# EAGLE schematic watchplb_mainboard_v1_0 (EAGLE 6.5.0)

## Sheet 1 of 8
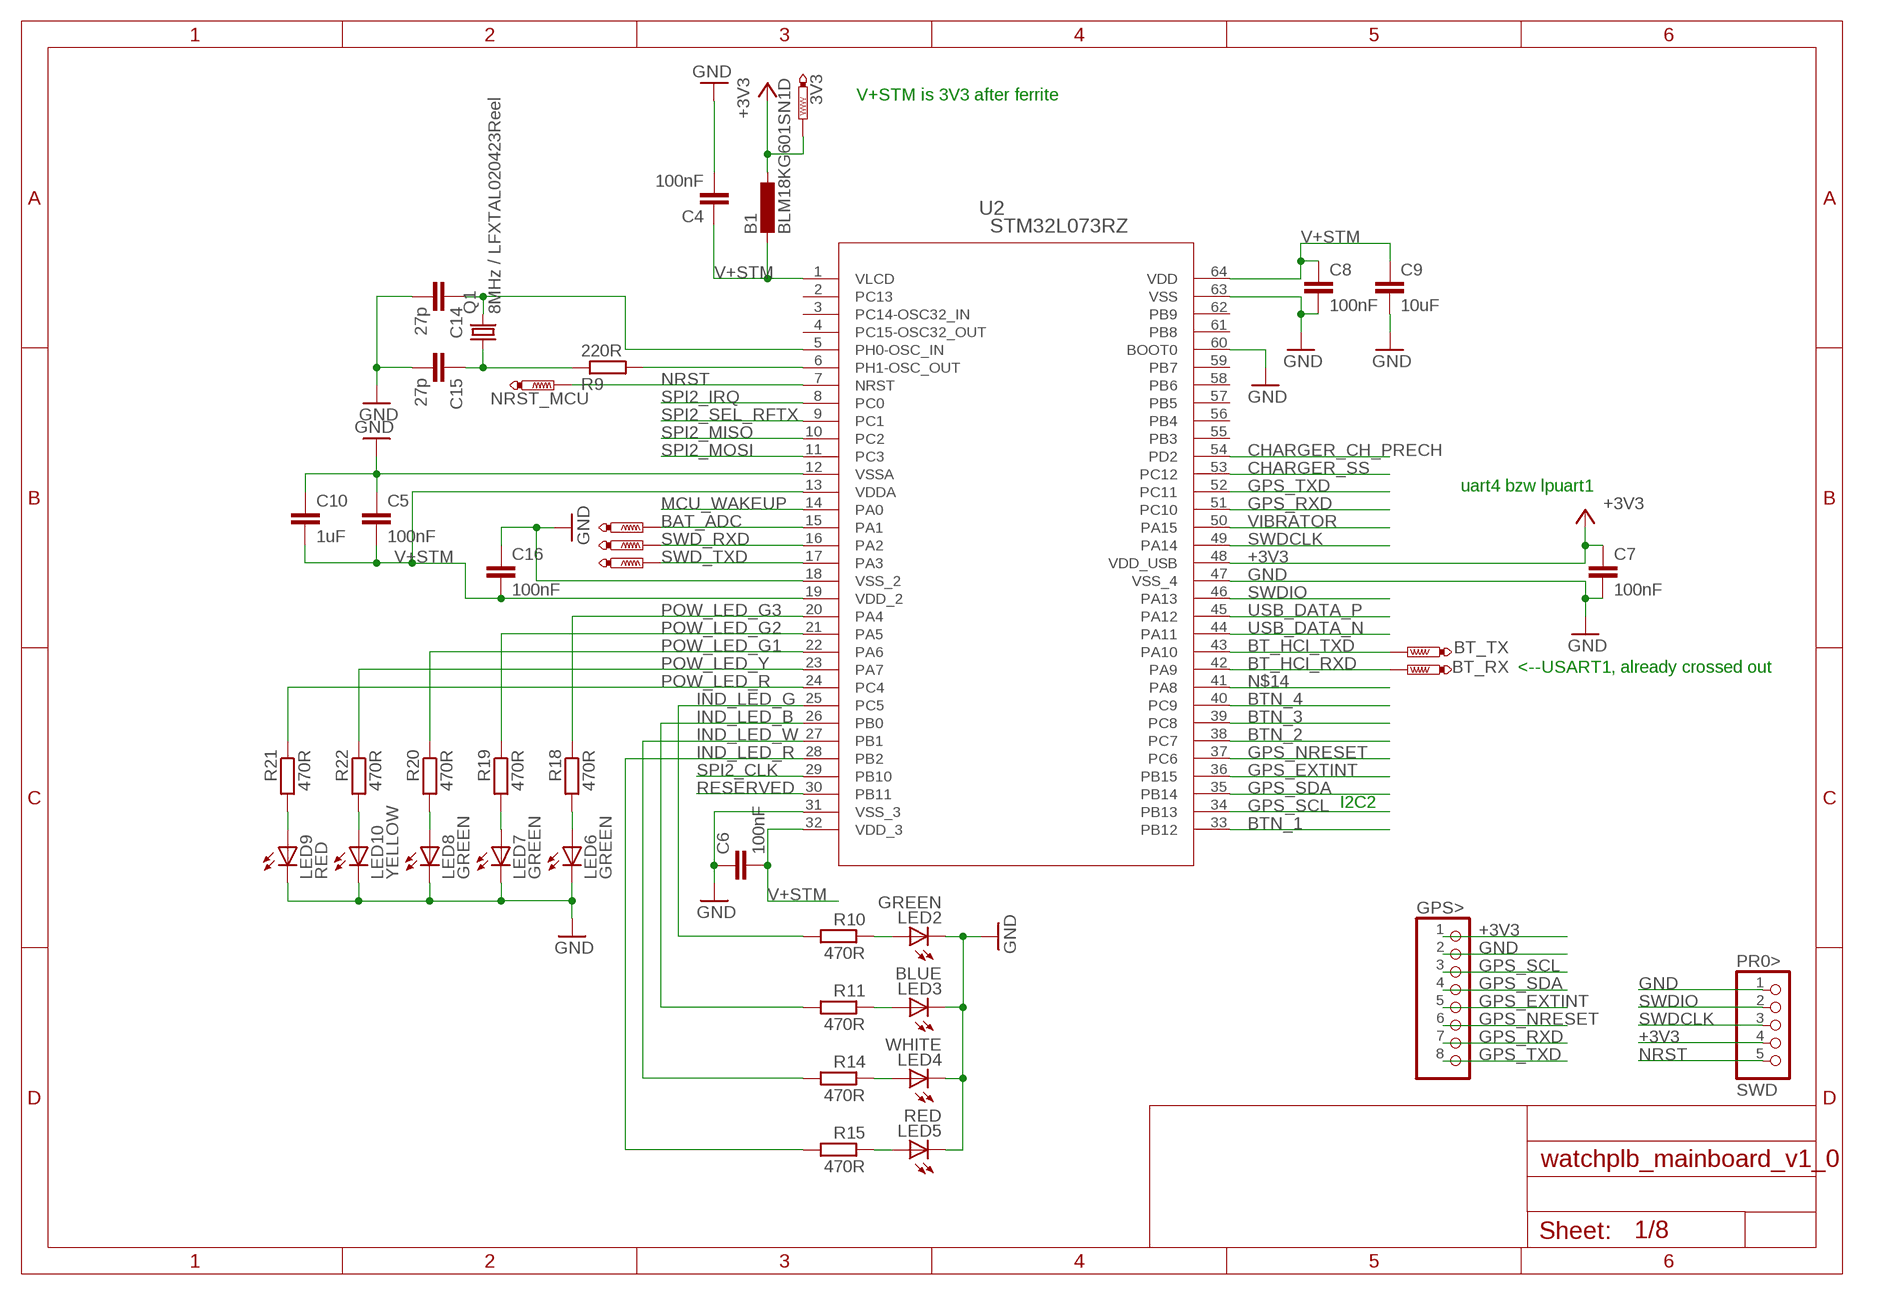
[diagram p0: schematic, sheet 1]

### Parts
3V3  PTR1B1,27  [B1,27]
B1  BLM18KG601SN1D  B-EU_B0603  [L0603]
BAT_ADC  PTR1B1,27  [B1,27]
BT_RX  PTR1B1,27  [B1,27]
BT_TX  PTR1B1,27  [B1,27]
C4  100nF  C-EUC0805  [C0805]
C5  100nF  C-EUC0805  [C0805]
C6  100nF  C-EUC0805  [C0805]
C7  100nF  C-EUC0805  [C0805]
C8  100nF  C-EUC0805  [C0805]
C9  10uF  C-EUC1206  [C1206]
C10  1uF  C-EUC0805  [C0805]
C14  27p  C-EUC0805  [C0805]
C15  27p  C-EUC0805  [C0805]
C16  100nF  C-EUC0805  [C0805]
GPS>  PINHD-1X8  [1X08]
LED2  GREEN  LEDCHIP-LED0805  [CHIP-LED0805]
LED3  BLUE  LEDCHIP-LED0805  [CHIP-LED0805]
LED4  WHITE  LEDCHIP-LED0805  [CHIP-LED0805]
LED5  RED  LEDCHIP-LED0805  [CHIP-LED0805]
LED6  GREEN  LEDCHIP-LED0805  [CHIP-LED0805]
LED7  GREEN  LEDCHIP-LED0805  [CHIP-LED0805]
LED8  GREEN  LEDCHIP-LED0805  [CHIP-LED0805]
LED9  RED  LEDCHIP-LED0805  [CHIP-LED0805]
LED10  YELLOW  LEDCHIP-LED0805  [CHIP-LED0805]
NRST_MCU  PTR1B1,27  [B1,27]
PR0>  SWD  PINHD-1X5  [1X05]
Q1  8MHz / LFXTAL020423Reel  CRYSTALHC49UP  [HC49UP]
R9  220R  R-EU_M0805  [M0805]
R10  470R  R-EU_M0805  [M0805]
R11  470R  R-EU_M0805  [M0805]
R14  470R  R-EU_M0805  [M0805]
R15  470R  R-EU_M0805  [M0805]
R18  470R  R-EU_M0805  [M0805]
R19  470R  R-EU_M0805  [M0805]
R20  470R  R-EU_M0805  [M0805]
R21  470R  R-EU_M0805  [M0805]
R22  470R  R-EU_M0805  [M0805]
SWD_RXD  PTR1B1,27  [B1,27]
SWD_TXD  PTR1B1,27  [B1,27]
U2  STM32L073RZ  STM32L0X3RL  [LQFP64-10X10MM]

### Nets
+3V3: 3V3.TP B1.1 C7.1 GPS>.1 PR0>.4 U2.48(VDD_USB) ; also sheet 2,3,4,5,6,8
BAT_ADC: BAT_ADC.TP U2.15(PA1) ; also sheet 8
BT_HCI_RXD: BT_RX.TP U2.42(PA9) ; also sheet 4
BT_HCI_TXD: BT_TX.TP U2.43(PA10) ; also sheet 4
BTN_1: U2.33(PB12) ; also sheet 3
BTN_2: U2.38(PC7) ; also sheet 3
BTN_3: U2.39(PC8) ; also sheet 3
BTN_4: U2.40(PC9) ; also sheet 3
CHARGER_CH_PRECH: U2.54(PD2) ; also sheet 5
CHARGER_SS: U2.53(PC12) ; also sheet 5
GND: C4.2 C5.1 C6.1 C7.2 C8.2 C9.2 C10.1 C14.2 C15.2 C16.1 GPS>.2 LED2.C LED3.C LED4.C LED5.C LED6.C LED7.C LED8.C LED9.C LED10.C PR0>.1 U2.12(VSSA) U2.18(VSS_2) U2.31(VSS_3) U2.47(VSS_4) U2.60(BOOT0) U2.63(VSS) ; also sheet 2,3,4,5,6,7,8
GPS_EXTINT: GPS>.5 U2.36(PB15)
GPS_NRESET: GPS>.6 U2.37(PC6)
GPS_RXD: GPS>.7 U2.51(PC10)
GPS_SCL: GPS>.3 U2.34(PB13)
GPS_SDA: GPS>.4 U2.35(PB14)
GPS_TXD: GPS>.8 U2.52(PC11)
IND_LED_B: R11.2 U2.26(PB0)
IND_LED_G: R10.2 U2.25(PC5)
IND_LED_R: R15.2 U2.28(PB2)
IND_LED_W: R14.2 U2.27(PB1)
MCU_WAKEUP: U2.14(PA0) ; also sheet 3
N$1: LED2.A R10.1
N$4: LED3.A R11.1
N$5: C15.1 Q1.1 R9.1
N$6: C14.1 Q1.2 U2.5(PH0-OSC_IN)
N$9: R9.2 U2.6(PH1-OSC_OUT)
N$12: LED4.A R14.1
N$13: LED9.A R21.2
N$14: U2.41(PA8)
N$16: LED5.A R15.1
N$19: LED6.A R18.2
N$22: LED7.A R19.2
N$24: LED10.A R22.2
N$25: LED8.A R20.2
NRST: NRST_MCU.TP PR0>.5 U2.7(NRST) ; also sheet 3
POW_LED_G1: R20.1 U2.22(PA6)
POW_LED_G2: R19.1 U2.21(PA5)
POW_LED_G3: R18.1 U2.20(PA4)
POW_LED_R: R21.1 U2.24(PC4)
POW_LED_Y: R22.1 U2.23(PA7)
RESERVED: U2.30(PB11)
SPI2_CLK: U2.29(PB10) ; also sheet 2
SPI2_IRQ: U2.8(PC0) ; also sheet 2
SPI2_MISO: U2.10(PC2) ; also sheet 2
SPI2_MOSI: U2.11(PC3) ; also sheet 2
SPI2_SEL_RFTX: U2.9(PC1) ; also sheet 2
SWD_RXD: SWD_RXD.TP U2.16(PA2)
SWD_TXD: SWD_TXD.TP U2.17(PA3)
SWDCLK: PR0>.3 U2.49(PA14)
SWDIO: PR0>.2 U2.46(PA13)
USB_DATA_N: U2.44(PA11) ; also sheet 6
USB_DATA_P: U2.45(PA12) ; also sheet 6
V+STM: B1.2 C4.1 C5.2 C6.2 C8.1 C9.1 C10.2 C16.2 U2.1(VLCD) U2.13(VDDA) U2.19(VDD_2) U2.32(VDD_3) U2.64(VDD)
VIBRATOR: U2.50(PA15) ; also sheet 3
Unconnected: U2.2(PC13) U2.3(PC14-OSC32_IN) U2.4(PC15-OSC32_OUT) U2.55(PB3) U2.56(PB4) U2.57(PB5) U2.58(PB6) U2.59(PB7) U2.61(PB8) U2.62(PB9)

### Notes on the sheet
- V+STM is 3V3 after ferrite
- uart4 bzw lpuart1
- <--USART1, already crossed out
- I2C2

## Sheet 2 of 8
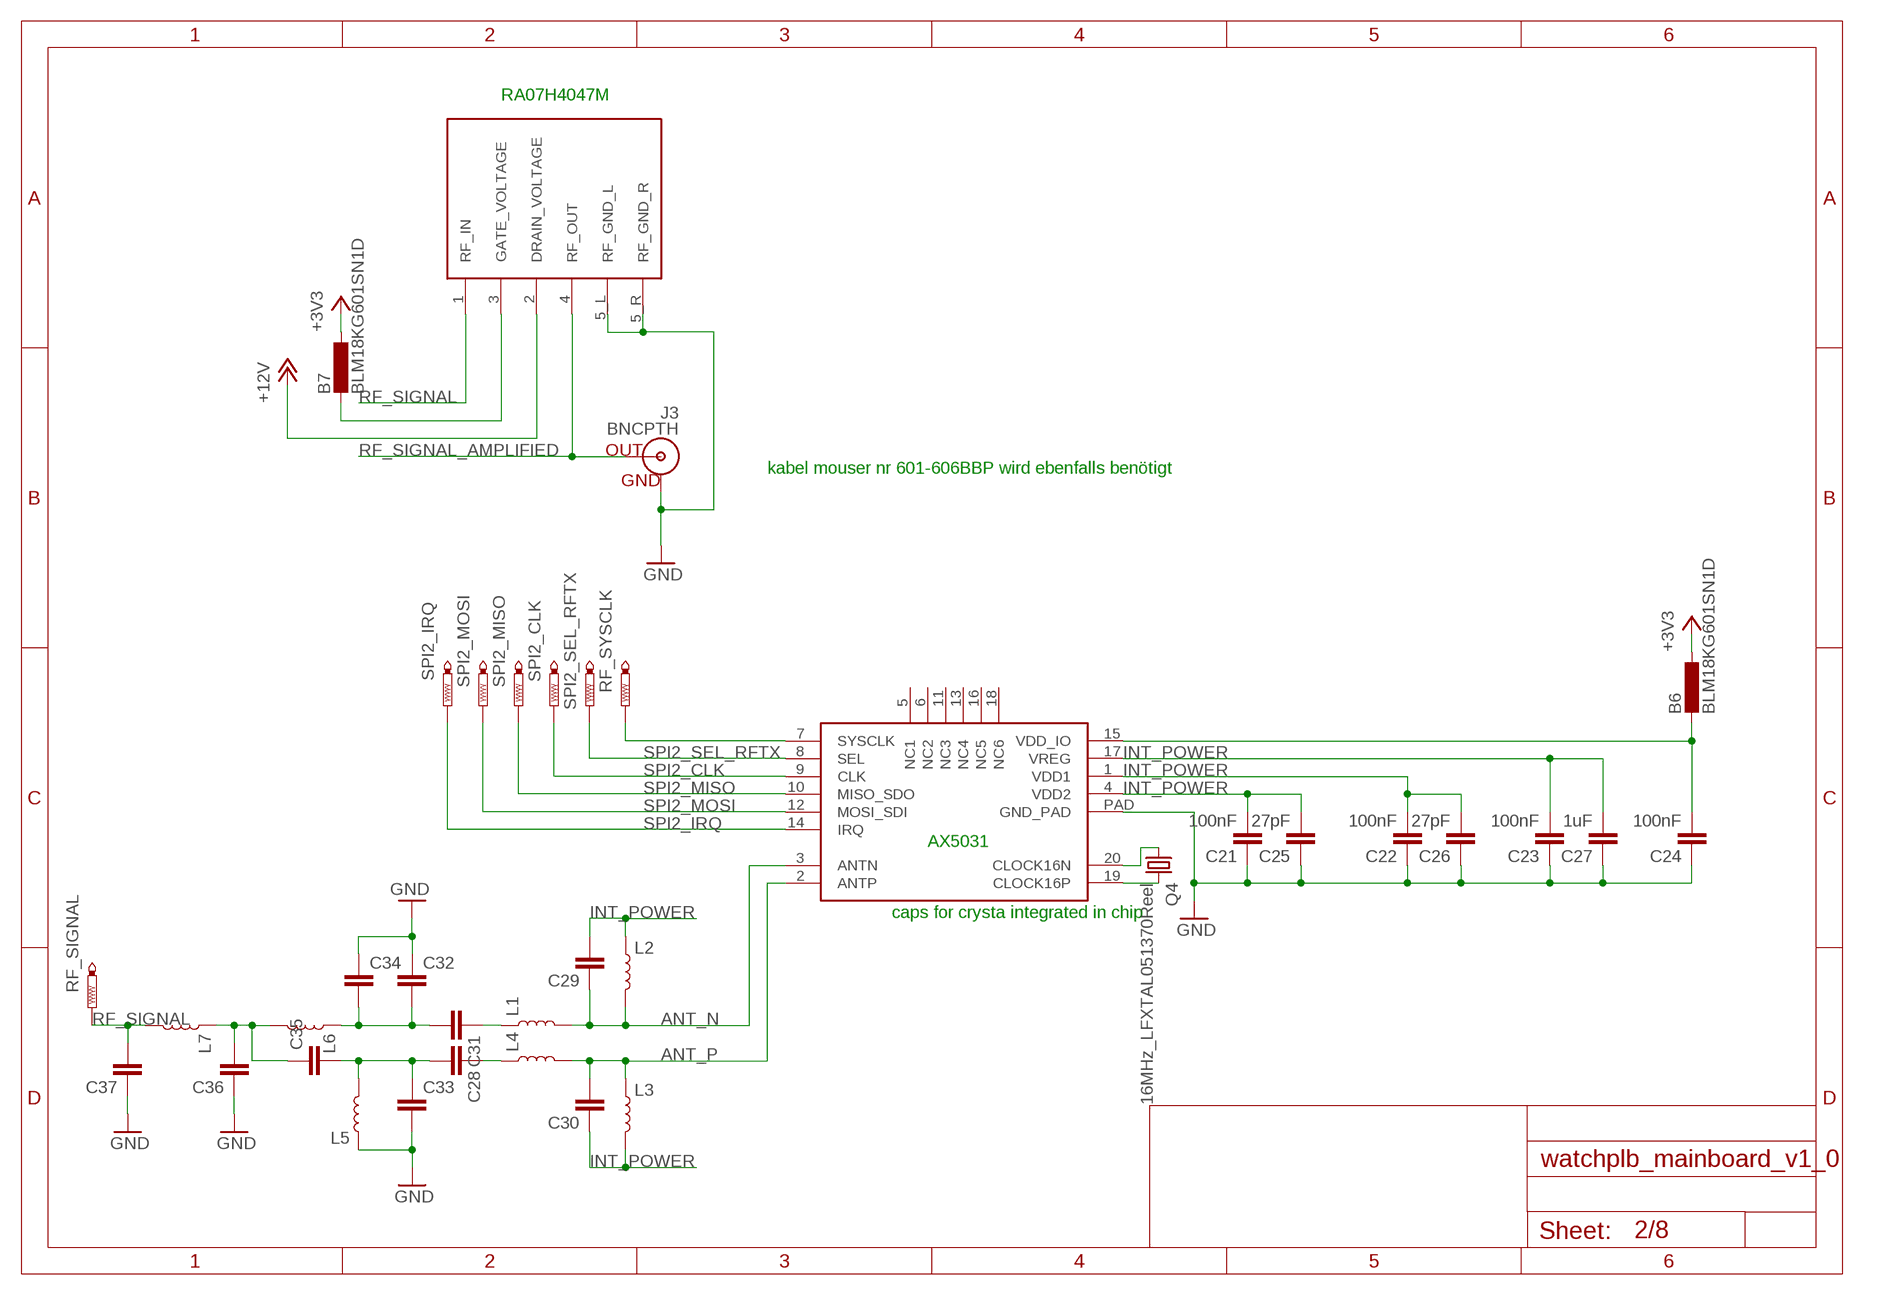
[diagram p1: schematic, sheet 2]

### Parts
B6  BLM18KG601SN1D  B-EU_B0603  [L0603]
B7  BLM18KG601SN1D  B-EU_B0603  [L0603]
C21  100nF  C-EUC0805  [C0805]
C22  100nF  C-EUC0805  [C0805]
C23  100nF  C-EUC0805  [C0805]
C24  100nF  C-EUC0805  [C0805]
C25  27pF  C-EUC0805  [C0805]
C26  27pF  C-EUC0805  [C0805]
C27  1uF  C-EUC0805  [C0805]
C28  C-EUC0805  [C0805]
C29  C-EUC0805  [C0805]
C30  C-EUC0805  [C0805]
C31  C-EUC0805  [C0805]
C32  C-EUC0805  [C0805]
C33  C-EUC0805  [C0805]
C34  C-EUC0805  [C0805]
C35  C-EUC0805  [C0805]
C36  C-EUC0805  [C0805]
C37  C-EUC0805  [C0805]
IC4  AX5031  [QFN20]
J3  BNCPTH  [BNC]
L1  INDUCTOR-0805-3.3UH  [0805]
L2  INDUCTOR-0805-3.3UH  [0805]
L3  INDUCTOR-0805-3.3UH  [0805]
L4  INDUCTOR-0805-3.3UH  [0805]
L5  INDUCTOR-0805-3.3UH  [0805]
L6  INDUCTOR-0805-3.3UH  [0805]
L7  INDUCTOR-0805-3.3UH  [0805]
Q4  16MHz_LFXTAL051370Reel  CRYSTALHC49UP  [HC49UP]
RF_SIGNAL  PTR1B2,54  [B2,54]
RF_SYSCLK  PTR1B1,27  [B1,27]
SPI2_CLK  PTR1B1,27  [B1,27]
SPI2_IRQ  PTR1B1,27  [B1,27]
SPI2_MISO  PTR1B1,27  [B1,27]
SPI2_MOSI  PTR1B1,27  [B1,27]
SPI2_SEL_RFTX  PTR1B1,27  [B1,27]
U$2  RA07H4047M  [RA07H4047M]

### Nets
+3V3: B6.1 B7.1 ; also sheet 1,3,4,5,6,8
+12V: U$2.2(DRAIN_VOLTAGE) ; also sheet 8
ANT_N: C29.1 IC4.3(ANTN) L1.2 L2.2
ANT_P: C30.2 IC4.2(ANTP) L3.1 L4.2
GND: C21.1 C22.1 C23.1 C24.1 C25.1 C26.1 C27.1 C32.1 C33.2 C34.1 C36.1 C37.1 IC4.PAD(GND_PAD) J3.GND L5.1 U$2.5_L(RF_GND_L) U$2.5_R(RF_GND_R) ; also sheet 1,3,4,5,6,7,8
INT_POWER: C21.2 C22.2 C23.2 C25.2 C26.2 C27.2 C29.2 C30.1 IC4.1(VDD1) IC4.4(VDD2) IC4.17(VREG) L2.1 L3.2
N$33: IC4.19(CLOCK16P) Q4.2
N$34: IC4.20(CLOCK16N) Q4.1
N$37: IC4.7(SYSCLK) RF_SYSCLK.TP
N$39: C28.1 L4.1
N$40: C31.1 L1.1
N$42: C31.2 C32.2 C34.2 L6.1
N$43: C28.2 C33.1 C35.2 L5.2
N$45: C35.1 C36.2 L6.2 L7.1
N$82: B6.2 C24.2 IC4.15(VDD_IO)
N$83: B7.2 U$2.3(GATE_VOLTAGE)
RF_SIGNAL: C37.2 L7.2 RF_SIGNAL.TP U$2.1(RF_IN)
RF_SIGNAL_AMPLIFIED: J3.S(OUT) U$2.4(RF_OUT)
SPI2_CLK: IC4.9(CLK) SPI2_CLK.TP ; also sheet 1
SPI2_IRQ: IC4.14(IRQ) SPI2_IRQ.TP ; also sheet 1
SPI2_MISO: IC4.10(MISO_SDO) SPI2_MISO.TP ; also sheet 1
SPI2_MOSI: IC4.12(MOSI_SDI) SPI2_MOSI.TP ; also sheet 1
SPI2_SEL_RFTX: IC4.8(SEL) SPI2_SEL_RFTX.TP ; also sheet 1
Unconnected: IC4.5(NC1) IC4.6(NC2) IC4.11(NC3) IC4.13(NC4) IC4.16(NC5) IC4.18(NC6)

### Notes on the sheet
- RA07H4047M
- kabel mouser nr 601-606BBP wird ebenfalls benötigt
- AX5031
- caps for crysta integrated in chip

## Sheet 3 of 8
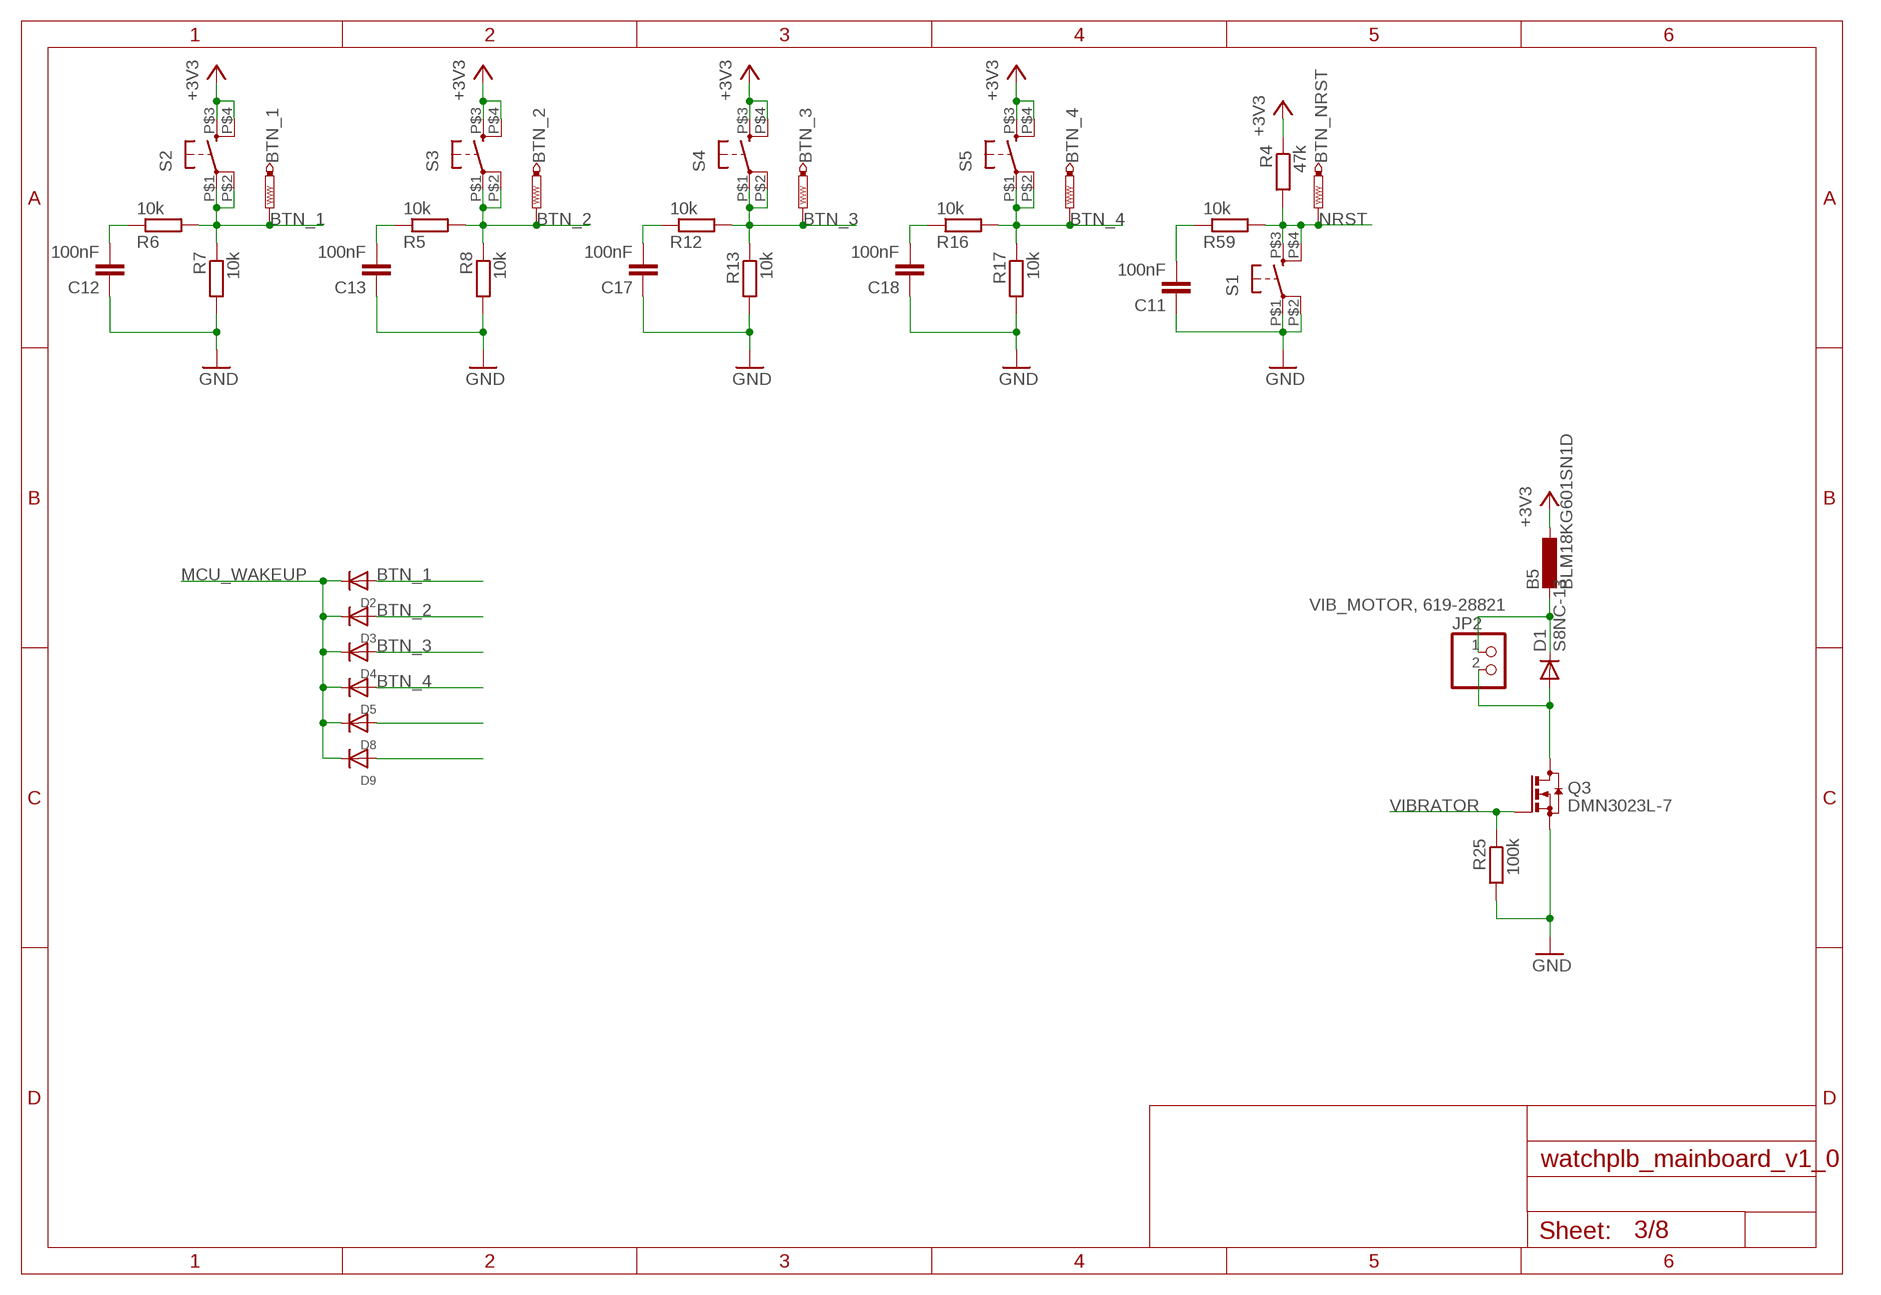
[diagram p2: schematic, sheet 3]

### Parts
B5  BLM18KG601SN1D  B-EU_B0603  [L0603]
BTN_1  PTR1B1,27  [B1,27]
BTN_2  PTR1B1,27  [B1,27]
BTN_3  PTR1B1,27  [B1,27]
BTN_4  PTR1B1,27  [B1,27]
BTN_NRST  PTR1B1,27  [B1,27]
C11  100nF  C-EUC0805  [C0805]
C12  100nF  C-EUC0805  [C0805]
C13  100nF  C-EUC0805  [C0805]
C17  100nF  C-EUC0805  [C0805]
C18  100nF  C-EUC0805  [C0805]
D1  S8NC-13  DIODE-SMC  [SMC]
D2  DIODESOD-123  [SOD-123]
D3  DIODESOD-123  [SOD-123]
D4  DIODESOD-123  [SOD-123]
D5  DIODESOD-123  [SOD-123]
D8  DIODESOD-123  [SOD-123]
D9  DIODESOD-123  [SOD-123]
JP2  VIB_MOTOR, 619-28821  PINHD-1X2  [1X02]
Q3  DMN3023L-7  BSS123  [SOT23]
R4  47k  R-EU_M0805  [M0805]
R5  10k  R-EU_M0805  [M0805]
R6  10k  R-EU_M0805  [M0805]
R7  10k  R-EU_M0805  [M0805]
R8  10k  R-EU_M0805  [M0805]
R12  10k  R-EU_M0805  [M0805]
R13  10k  R-EU_M0805  [M0805]
R16  10k  R-EU_M0805  [M0805]
R17  10k  R-EU_M0805  [M0805]
R25  100k  R-EU_M0805  [M0805]
R59  10k  R-EU_M0805  [M0805]
S1  TL3305  [SMD_SWITCH]
S2  TL3305  [SMD_SWITCH]
S3  TL3305  [SMD_SWITCH]
S4  TL3305  [SMD_SWITCH]
S5  TL3305  [SMD_SWITCH]

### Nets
+3V3: B5.1 R4.1 S2.P$3(S) S2.P$4(S1) S3.P$3(S) S3.P$4(S1) S4.P$3(S) S4.P$4(S1) S5.P$3(S) S5.P$4(S1) ; also sheet 1,2,4,5,6,8
BTN_1: BTN_1.TP D2.A R6.2 R7.1 S2.P$1(P) S2.P$2(P1) ; also sheet 1
BTN_2: BTN_2.TP D3.A R5.2 R8.1 S3.P$1(P) S3.P$2(P1) ; also sheet 1
BTN_3: BTN_3.TP D4.A R12.2 R13.1 S4.P$1(P) S4.P$2(P1) ; also sheet 1
BTN_4: BTN_4.TP D5.A R16.2 R17.1 S5.P$1(P) S5.P$2(P1) ; also sheet 1
GND: C11.1 C12.1 C13.1 C17.1 C18.1 Q3.2(S) R7.2 R8.2 R13.2 R17.2 R25.2 S1.P$1(P) S1.P$2(P1) ; also sheet 1,2,4,5,6,7,8
MCU_WAKEUP: D2.C D3.C D4.C D5.C D8.C D9.C ; also sheet 1
N$2: C12.2 R6.1
N$7: C13.2 R5.1
N$11: C17.2 R12.1
N$18: C18.2 R16.1
N$28: D1.A JP2.2 Q3.3(D)
N$67: D8.A
N$68: D9.A
N$81: B5.2 D1.C JP2.1
N$86: C11.2 R59.1
NRST: BTN_NRST.TP R4.2 R59.2 S1.P$3(S) S1.P$4(S1) ; also sheet 1
VIBRATOR: Q3.1(G) R25.1 ; also sheet 1

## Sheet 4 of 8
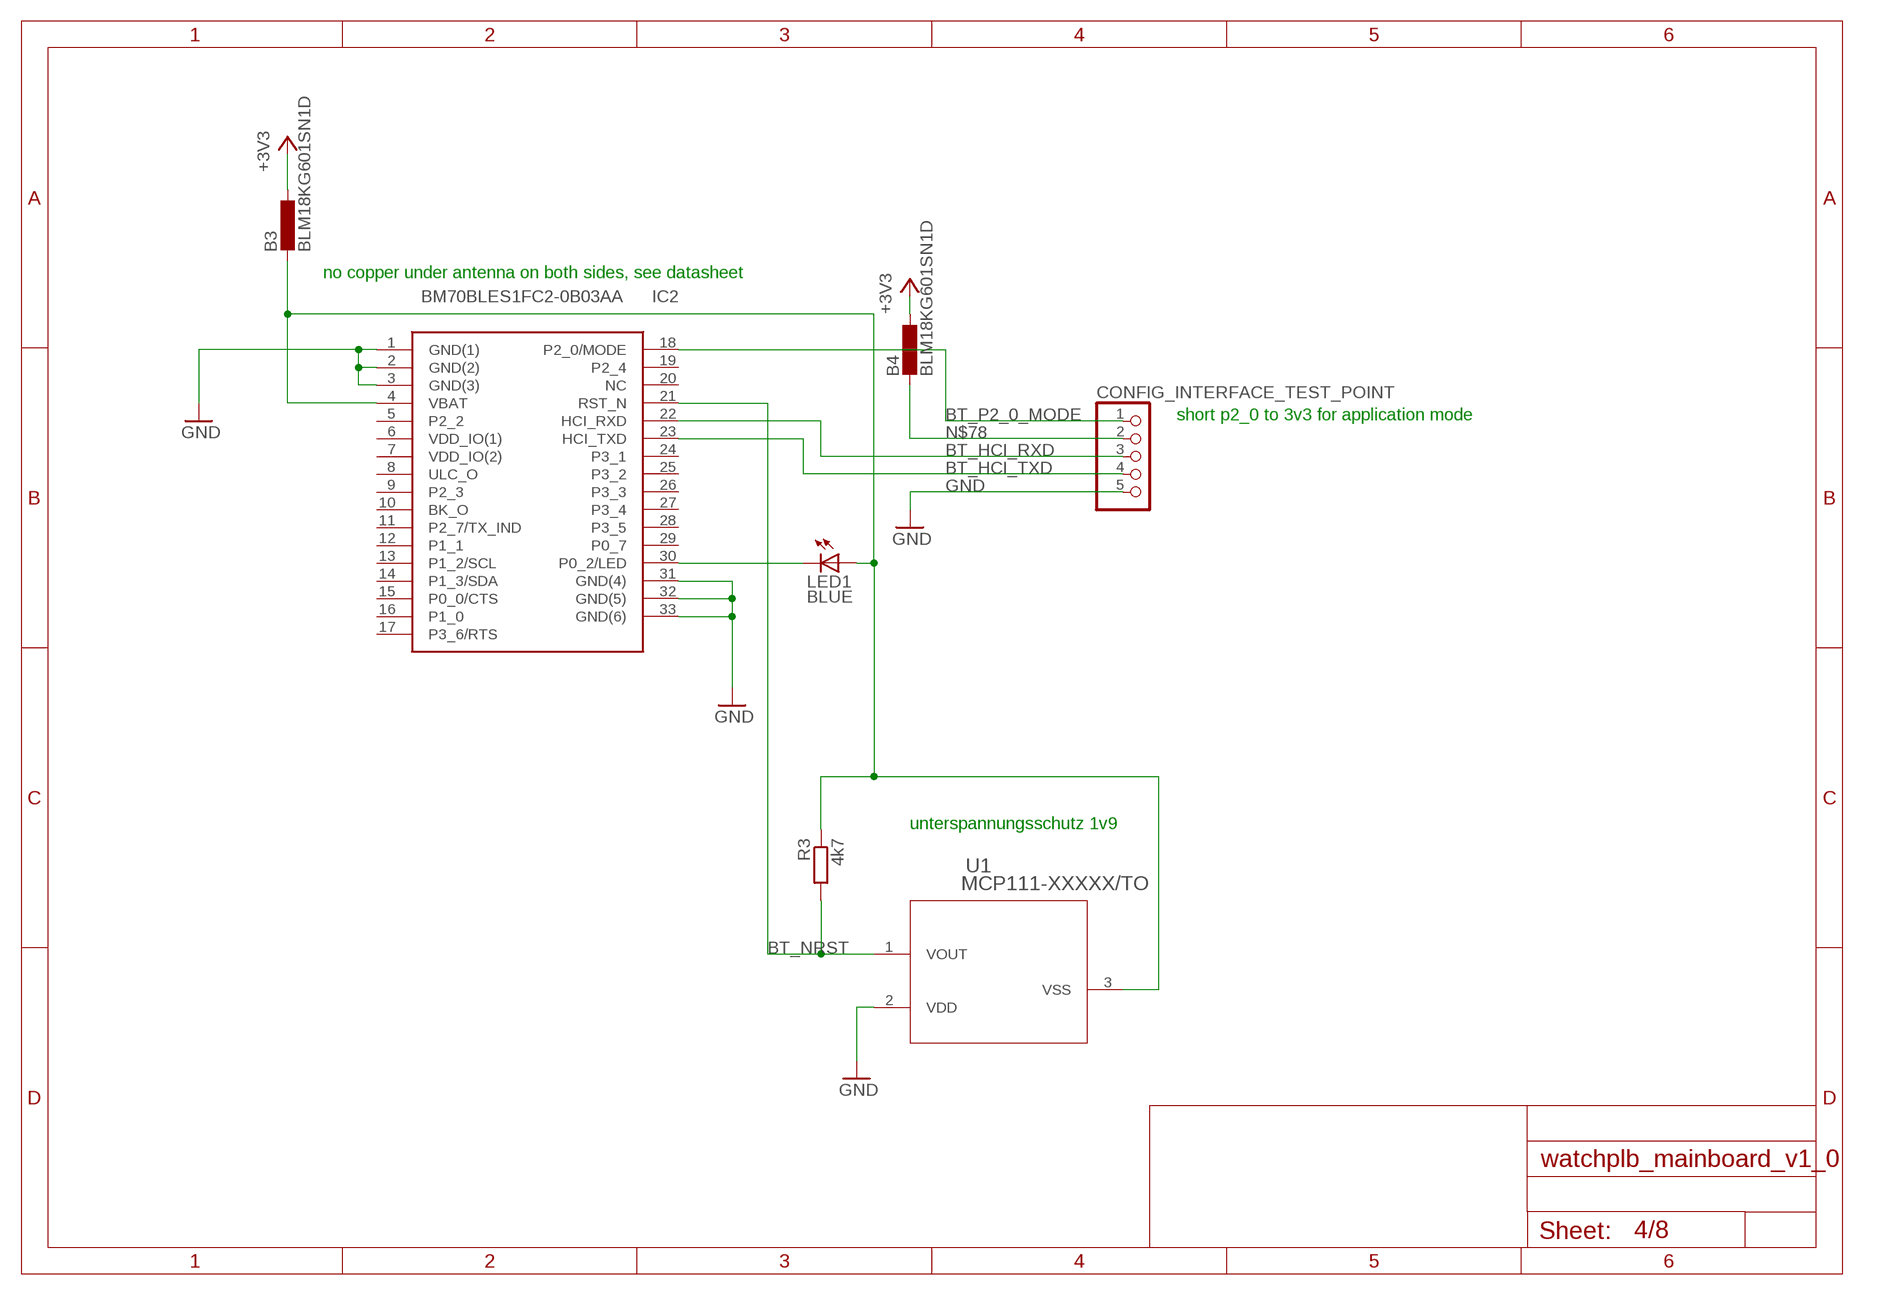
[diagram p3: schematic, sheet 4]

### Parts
B3  BLM18KG601SN1D  B-EU_B0603  [L0603]
B4  BLM18KG601SN1D  B-EU_B0603  [L0603]
CONFIG_INTERFACE_TEST_POINT  PINHD-1X5  [1X05]
IC2  BM70BLES1FC2-0B03AA  [BM78SPPS5NC2_1]
LED1  BLUE  LEDCHIP-LED0805  [CHIP-LED0805]
R3  4k7  R-EU_M0805  [M0805]
U1  MCP111-XXXXX/TO  [TO-92_MC]

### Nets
+3V3: B3.1 B4.1 ; also sheet 1,2,3,5,6,8
BT_HCI_RXD: CONFIG_INTERFACE_TEST_POINT.3 IC2.22(HCI_RXD) ; also sheet 1
BT_HCI_TXD: CONFIG_INTERFACE_TEST_POINT.4 IC2.23(HCI_TXD) ; also sheet 1
BT_NRST: IC2.21(RST_N) R3.2 U1.1(VOUT)
BT_P2_0_MODE: CONFIG_INTERFACE_TEST_POINT.1 IC2.18(P2_0/MODE)
GND: CONFIG_INTERFACE_TEST_POINT.5 IC2.1(GND(1)) IC2.2(GND(2)) IC2.3(GND(3)) IC2.31(GND(4)) IC2.32(GND(5)) IC2.33(GND(6)) U1.2(VDD) ; also sheet 1,2,3,5,6,7,8
N$3: IC2.30(P0_2/LED) LED1.C
N$78: B4.2 CONFIG_INTERFACE_TEST_POINT.2
N$80: B3.2 IC2.4(VBAT) LED1.A R3.1 U1.3(VSS)
Unconnected: IC2.5(P2_2) IC2.6(VDD_IO(1)) IC2.7(VDD_IO(2)) IC2.8(ULC_O) IC2.9(P2_3) IC2.10(BK_O) IC2.11(P2_7/TX_IND) IC2.12(P1_1) IC2.13(P1_2/SCL) IC2.14(P1_3/SDA) IC2.15(P0_0/CTS) IC2.16(P1_0) IC2.17(P3_6/RTS) IC2.19(P2_4) IC2.20(NC) IC2.24(P3_1) IC2.25(P3_2) IC2.26(P3_3) IC2.27(P3_4) IC2.28(P3_5) IC2.29(P0_7)

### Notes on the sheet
- no copper under antenna on both sides, see datasheet
- short p2_0 to 3v3 for application mode
- unterspannungsschutz 1v9

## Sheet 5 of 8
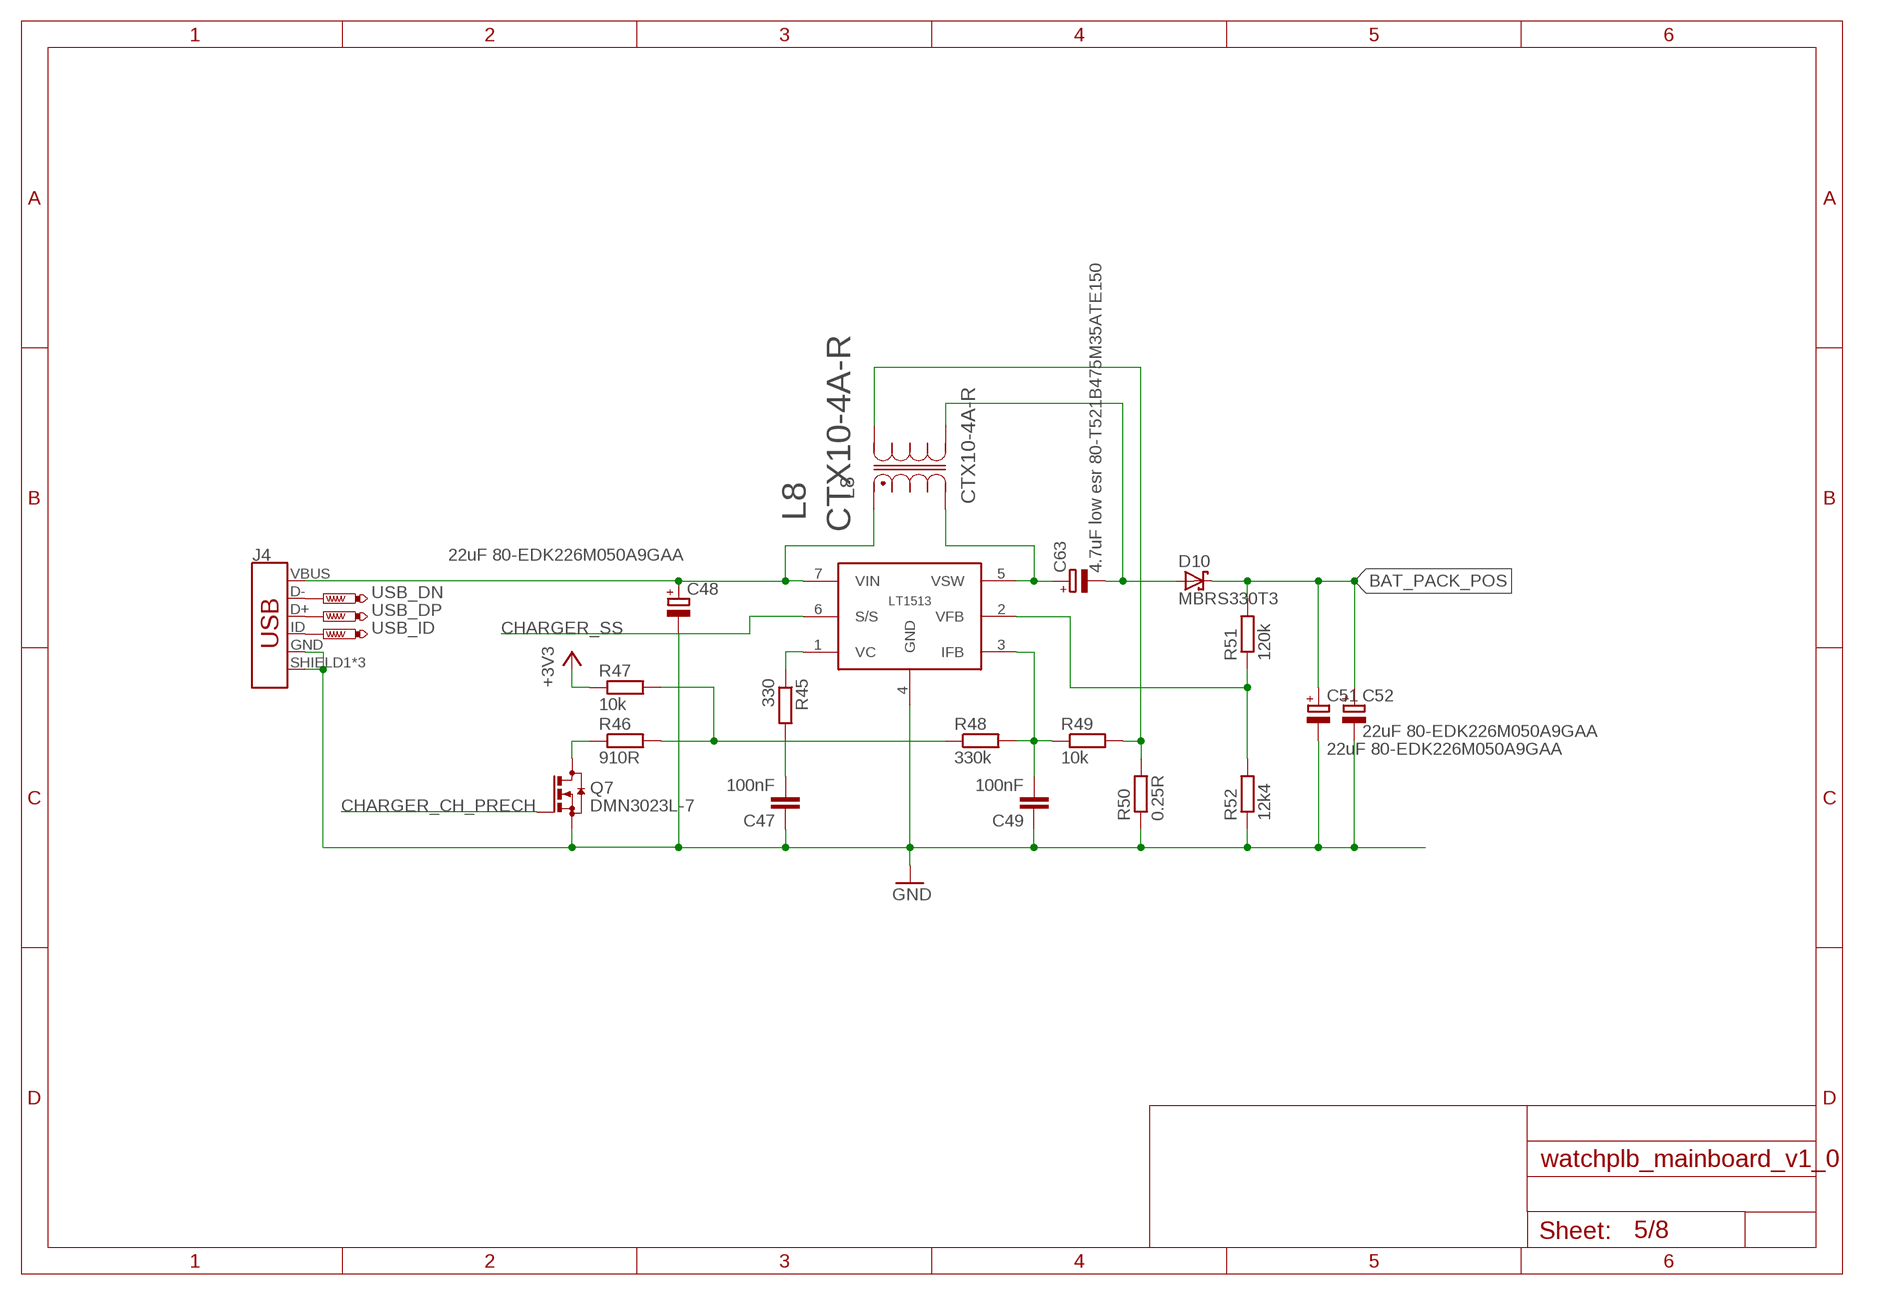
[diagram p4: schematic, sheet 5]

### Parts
C47  100nF  C-EUC0805K  [C0805K]
C48  22uF 80-EDK226M050A9GAA  CPOL-EUE  [PANASONIC_E]
C49  100nF  C-EUC0805K  [C0805K]
C51  22uF 80-EDK226M050A9GAA  CPOL-EUE  [PANASONIC_E]
C52  22uF 80-EDK226M050A9GAA  CPOL-EUE  [PANASONIC_E]
C63  4.7uF low esr 80-T521B475M35ATE150  CPOL-EUB/3528-21R  [B/3528-21R]
D10  MBRS330T3  [SMC]
IC1  LT1513  [TO220-7]
J4  USB_MICRO-B_FEMALE-SMT  [USB-B-MICRO-SMD]
L8  CTX10-4A-R  [INDM115115X635N]
Q7  DMN3023L-7  BSS123  [SOT23]
R45  330  R-EU_M0805  [M0805]
R46  910R  R-EU_M0805  [M0805]
R47  10k  R-EU_M0805  [M0805]
R48  330k  R-EU_M0805  [M0805]
R49  10k  R-EU_M0805  [M0805]
R50  0.25R  R-EU_R2512  [R2512]
R51  120k  R-EU_M0805  [M0805]
R52  12k4  R-EU_M0805  [M0805]
USB_DN  PTR1B1,27  [B1,27]
USB_DP  PTR1B1,27  [B1,27]
USB_ID  PTR1B1,27  [B1,27]

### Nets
+3V3: R47.1 ; also sheet 1,2,3,4,6,8
BAT_PACK_POS: C51.+ C52.+ D10.C R51.2 ; also sheet 7,8
CHARGER_CH_PRECH: Q7.1(G) ; also sheet 1
CHARGER_SS: IC1.6(S/S) ; also sheet 1
GND: C47.1 C48.- C49.1 C51.- C52.- IC1.4(GND) J4.GND J4.SHIELD1(SHIELD) J4.SHIELD2(SHIELD) J4.SHIELD3(SHIELD) Q7.2(S) R50.1 R52.1 ; also sheet 1,2,3,4,6,7,8
N$61: C63.+ IC1.5(VSW) L8.2
N$69: C48.+ IC1.7(VIN) J4.VBUS L8.1
N$70: L8.4 R49.2 R50.2
N$71: C47.2 R45.2
N$72: IC1.1(VC) R45.1
N$73: Q7.3(D) R46.1
N$74: R46.2 R47.2 R48.1
N$76: C49.2 IC1.3(IFB) R48.2 R49.1
N$77: IC1.2(VFB) R51.1 R52.2
N$87: J4.ID USB_ID.TP
N$88: J4.D+ USB_DP.TP
N$90: J4.D- USB_DN.TP
N$91: C63.- D10.A L8.3

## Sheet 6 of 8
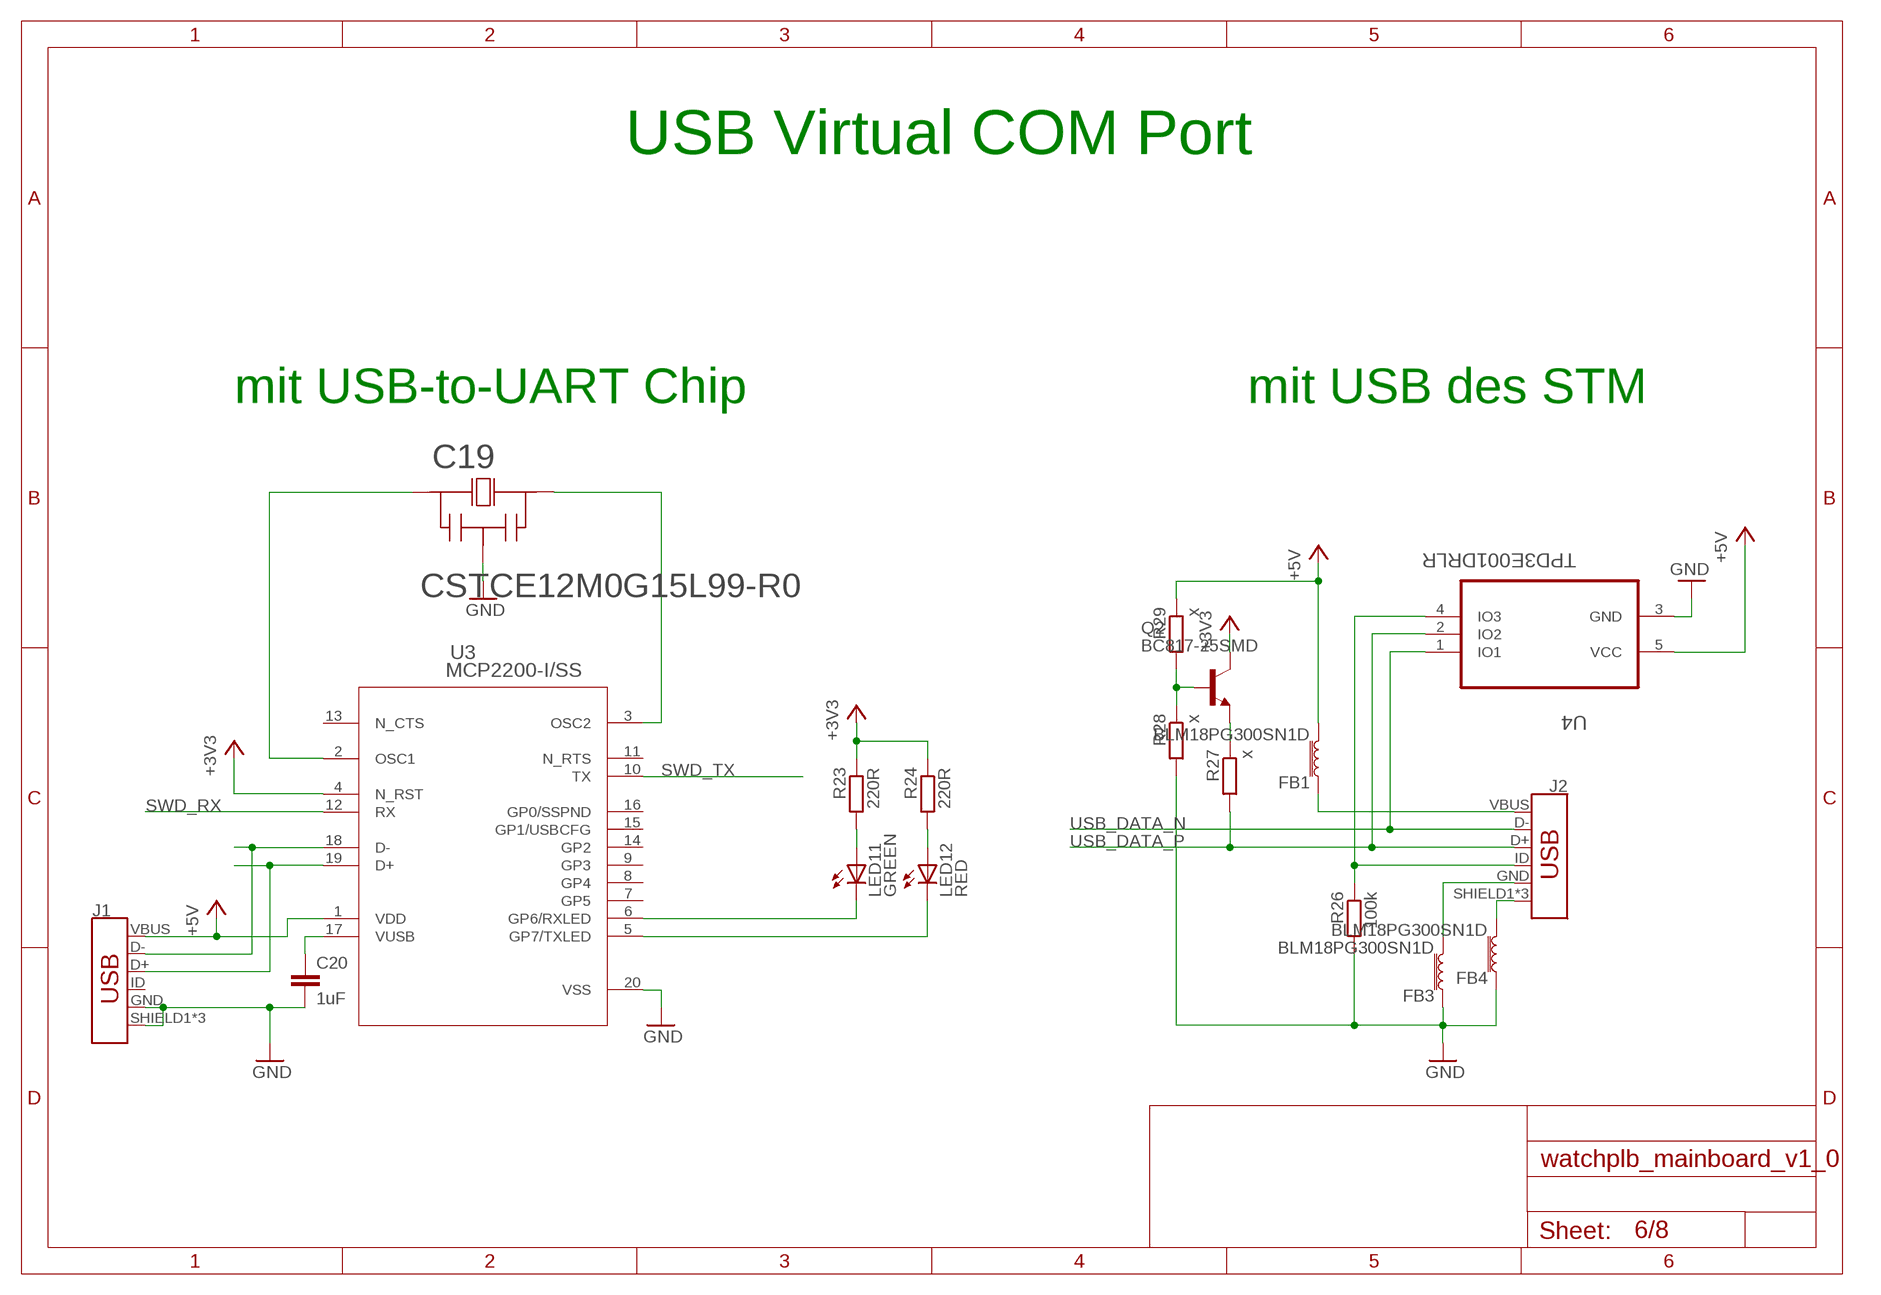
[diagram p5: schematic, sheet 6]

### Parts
C19  CSTCE12M0G15L99-R0  CSTCE8M00G52-R0  [CSTCE]
C20  1uF  C-EUC0805  [C0805]
FB1  BLM18PG300SN1D  FERRITE_BEAD-0603  [0603]
FB3  BLM18PG300SN1D  FERRITE_BEAD-0603  [0603]
FB4  BLM18PG300SN1D  FERRITE_BEAD-0603  [0603]
J1  USB_MICRO-B_FEMALE-SMT  [USB-B-MICRO-SMD]
J2  USB_MICRO-B_FEMALE-SMT  [USB-B-MICRO-SMD]
LED11  GREEN  LEDCHIP-LED0805  [CHIP-LED0805]
LED12  RED  LEDCHIP-LED0805  [CHIP-LED0805]
Q2  BC817-25SMD  [SOT23-BEC]
R23  220R  R-EU_M0805  [M0805]
R24  220R  R-EU_M0805  [M0805]
R26  100k  R-EU_M0805  [M0805]
R27  x  R-EU_M0805  [M0805]
R28  x  R-EU_M0805  [M0805]
R29  x  R-EU_M0805  [M0805]
U3  MCP2200-I/SS  [SSOP20_MC]
U4  TPD3E001DRLR  [SOT50P160X60-5N]

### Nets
+3V3: Q2.C R23.1 R24.1 U3.4(N_RST) ; also sheet 1,2,3,4,5,8
+5V: FB1.2 J1.VBUS R29.1 U3.1(VDD) U4.5(VCC)
GND: C19.2 C20.2 FB3.1 FB4.1 J1.GND J1.SHIELD1(SHIELD) J1.SHIELD2(SHIELD) J1.SHIELD3(SHIELD) R26.2 R28.2 U3.20(VSS) U4.3(GND) ; also sheet 1,2,3,4,5,7,8
N$8: LED11.A R23.2
N$10: C19.3 U3.3(OSC2)
N$15: C19.1 U3.2(OSC1)
N$17: J1.D- U3.18(D-)
N$20: J1.D+ U3.19(D+)
N$21: C20.1 U3.17(VUSB)
N$23: LED12.A R24.2
N$26: LED11.C U3.6(GP6/RXLED)
N$27: LED12.C U3.5(GP7/TXLED)
N$29: FB4.2 J2.SHIELD1(SHIELD) J2.SHIELD2(SHIELD) J2.SHIELD3(SHIELD)
N$30: FB3.2 J2.GND
N$31: FB1.1 J2.VBUS
N$32: J2.ID R26.1 U4.4(IO3)
N$35: Q2.E R27.1
N$36: Q2.B R28.1 R29.2
SWD_RX: U3.12(RX)
SWD_TX: U3.10(TX)
USB_DATA_N: J2.D- U4.1(IO1) ; also sheet 1
USB_DATA_P: J2.D+ R27.2 U4.2(IO2) ; also sheet 1
Unconnected: J1.ID U3.7(GP5) U3.8(GP4) U3.9(GP3) U3.11(N_RTS) U3.13(N_CTS) U3.14(GP2) U3.15(GP1/USBCFG) U3.16(GP0/SSPND)

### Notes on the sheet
- USB Virtual COM Port
- mit USB-to-UART Chip | mit USB des STM

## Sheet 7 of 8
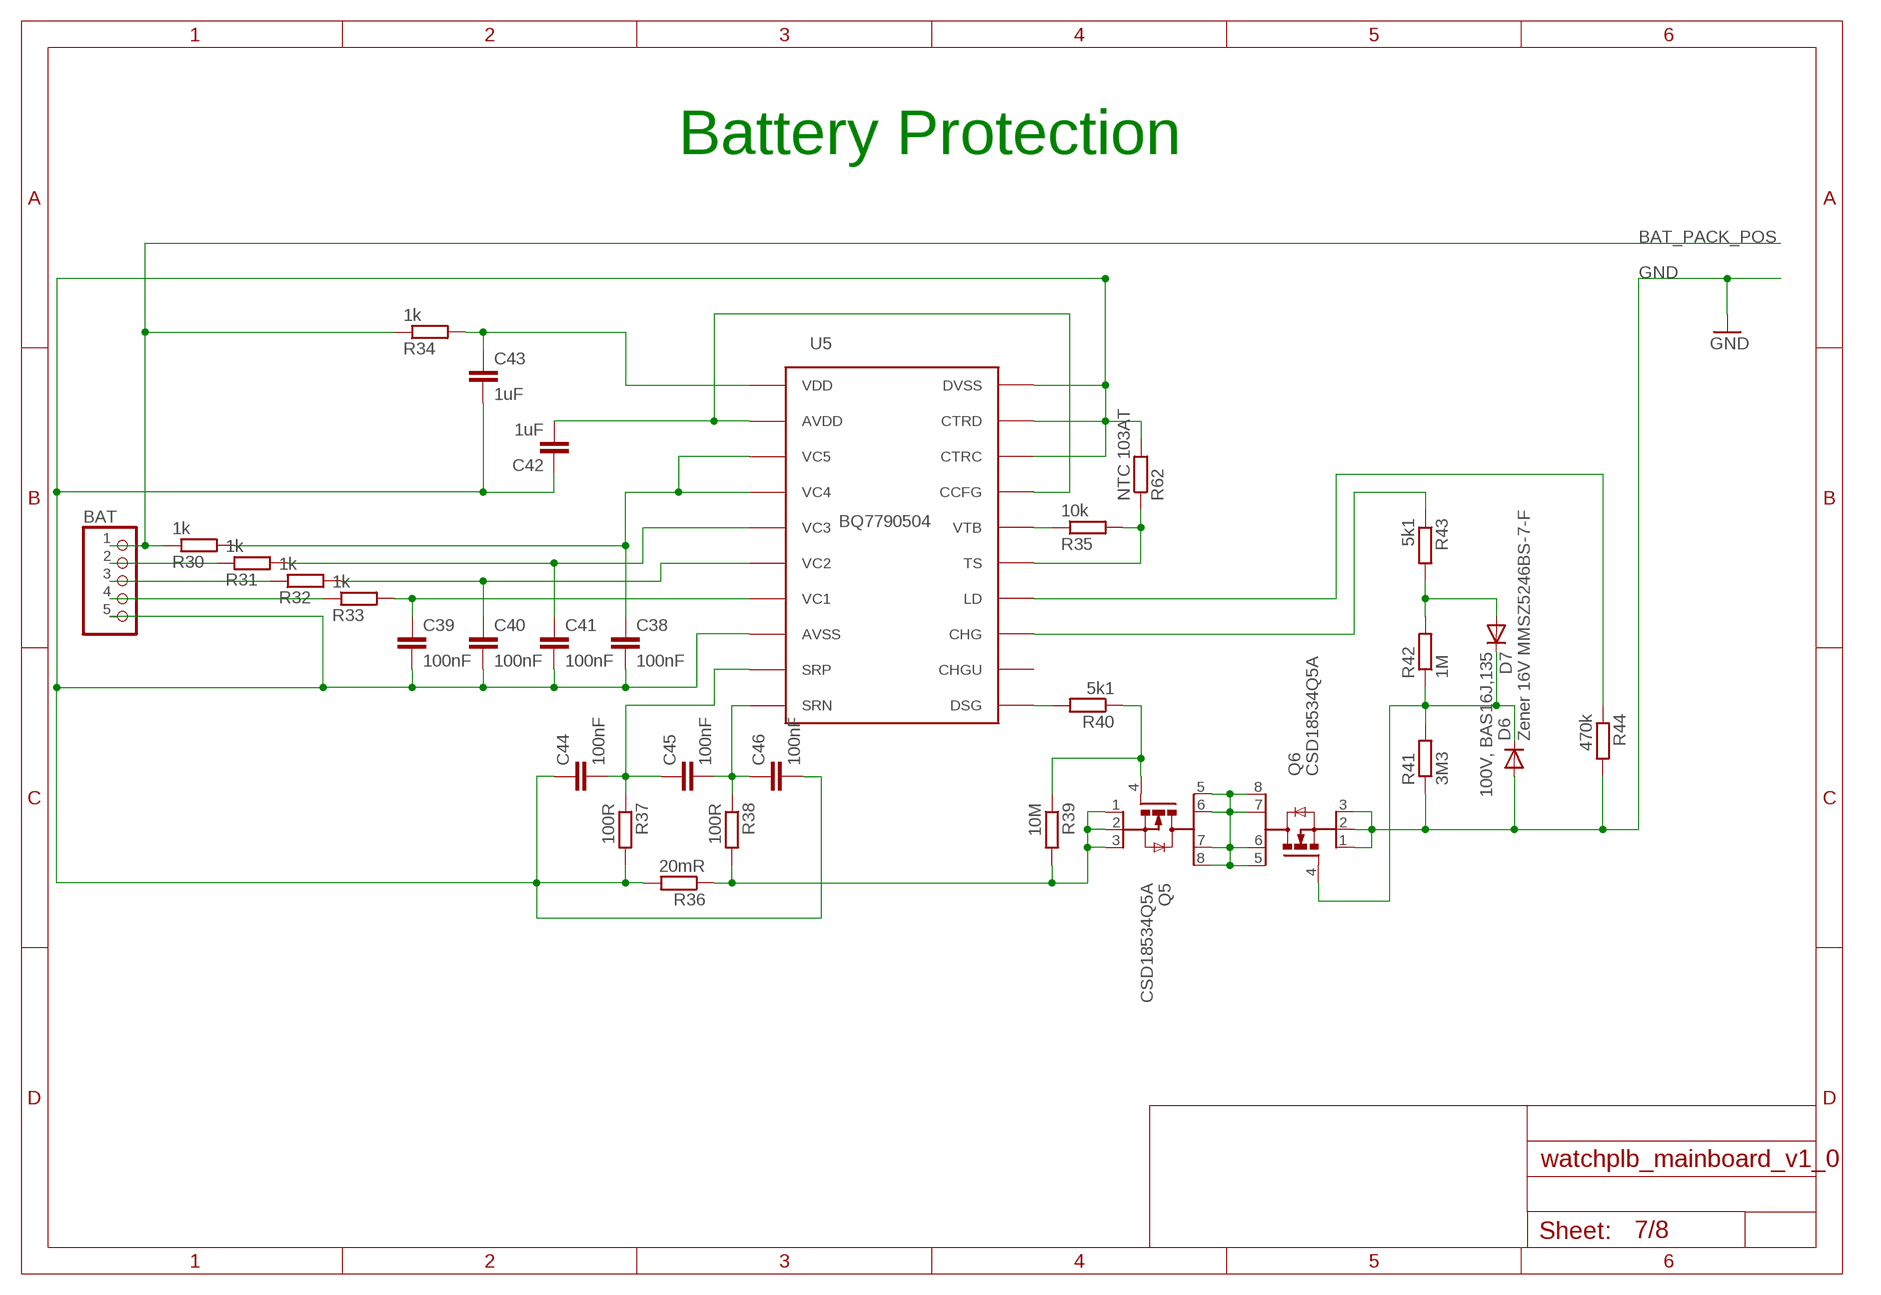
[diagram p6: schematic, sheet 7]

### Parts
BAT  PINHD-1X5  [1X05]
C38  100nF  C-EUC0805K  [C0805K]
C39  100nF  C-EUC0805K  [C0805K]
C40  100nF  C-EUC0805K  [C0805K]
C41  100nF  C-EUC0805K  [C0805K]
C42  1uF  C-EUC0805K  [C0805K]
C43  1uF  C-EUC0805K  [C0805K]
C44  100nF  C-EUC0805K  [C0805K]
C45  100nF  C-EUC0805K  [C0805K]
C46  100nF  C-EUC0805K  [C0805K]
D6  Zener 16V MMSZ5246BS-7-F  DIODE-SOD323-R  [SOD323-R]
D7  100V, BAS16J,135  DIODE-SOD323-R  [SOD323-R]
Q5  CSD18534Q5A  [TRANS_CSD18534Q5A]
Q6  CSD18534Q5A  [TRANS_CSD18534Q5A]
R30  1k  R-EU_M0805  [M0805]
R31  1k  R-EU_M0805  [M0805]
R32  1k  R-EU_M0805  [M0805]
R33  1k  R-EU_M0805  [M0805]
R34  1k  R-EU_M0805  [M0805]
R35  10k  R-EU_M0805  [M0805]
R36  20mR  R-EU_R2512  [R2512]
R37  100R  R-EU_M0805  [M0805]
R38  100R  R-EU_M0805  [M0805]
R39  10M  R-EU_M0805  [M0805]
R40  5k1  R-EU_M0805  [M0805]
R41  3M3  R-EU_M0805  [M0805]
R42  1M  R-EU_M0805  [M0805]
R43  5k1  R-EU_M0805  [M0805]
R44  470k  R-EU_M0805  [M0805]
R62  NTC 103AT  R-EU_M0805  [M0805]
U5  BQ7790504  BQ77904  [TSSOP-20/6MM]

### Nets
BAT_PACK_GND: BAT.5 C38.2 C39.2 C40.2 C41.2 C42.1 C43.2 C44.1 C46.2 R36.2 R37.2 R62.2 U5.8(AVSS) U5.18(CTRC) U5.19(CTRD) U5.20(DVSS)
BAT_PACK_POS: BAT.1 R30.1 R34.1 ; also sheet 5,8
GND: D6.A Q6.1 Q6.2 Q6.3 R41.1 R44.2 ; also sheet 1,2,3,4,5,6,8
N$38: R35.2 R62.1 U5.15(TS)
N$46: D6.C D7.C Q6.4 R41.2 R42.1
N$47: BAT.2 R31.1
N$48: BAT.3 R32.1
N$49: BAT.4 R33.1
N$50: C39.1 R33.2 U5.7(VC1)
N$51: C40.1 R32.2 U5.6(VC2)
N$52: C41.1 R31.2 U5.5(VC3)
N$53: C38.1 R30.2 U5.3(VC5) U5.4(VC4)
N$54: C43.1 R34.2 U5.1(VDD)
N$55: Q5.1 Q5.2 Q5.3 R36.1 R38.2 R39.2
N$56: C42.2 U5.2(AVDD) U5.17(CCFG)
N$57: C45.2 C46.1 R38.1 U5.10(SRN)
N$58: C44.2 C45.1 R37.1 U5.9(SRP)
N$59: Q5.5 Q5.6 Q5.7 Q5.8 Q6.5 Q6.6 Q6.7 Q6.8
N$60: R35.1 U5.16(VTB)
N$62: Q5.4 R39.1 R40.1
N$63: R40.2 U5.11(DSG)
N$64: D7.A R42.2 R43.2
N$65: R43.1 U5.13(CHG)
N$66: R44.1 U5.14(LD)
Unconnected: U5.12(CHGU)

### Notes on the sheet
- Battery Protection
- BQ7790504

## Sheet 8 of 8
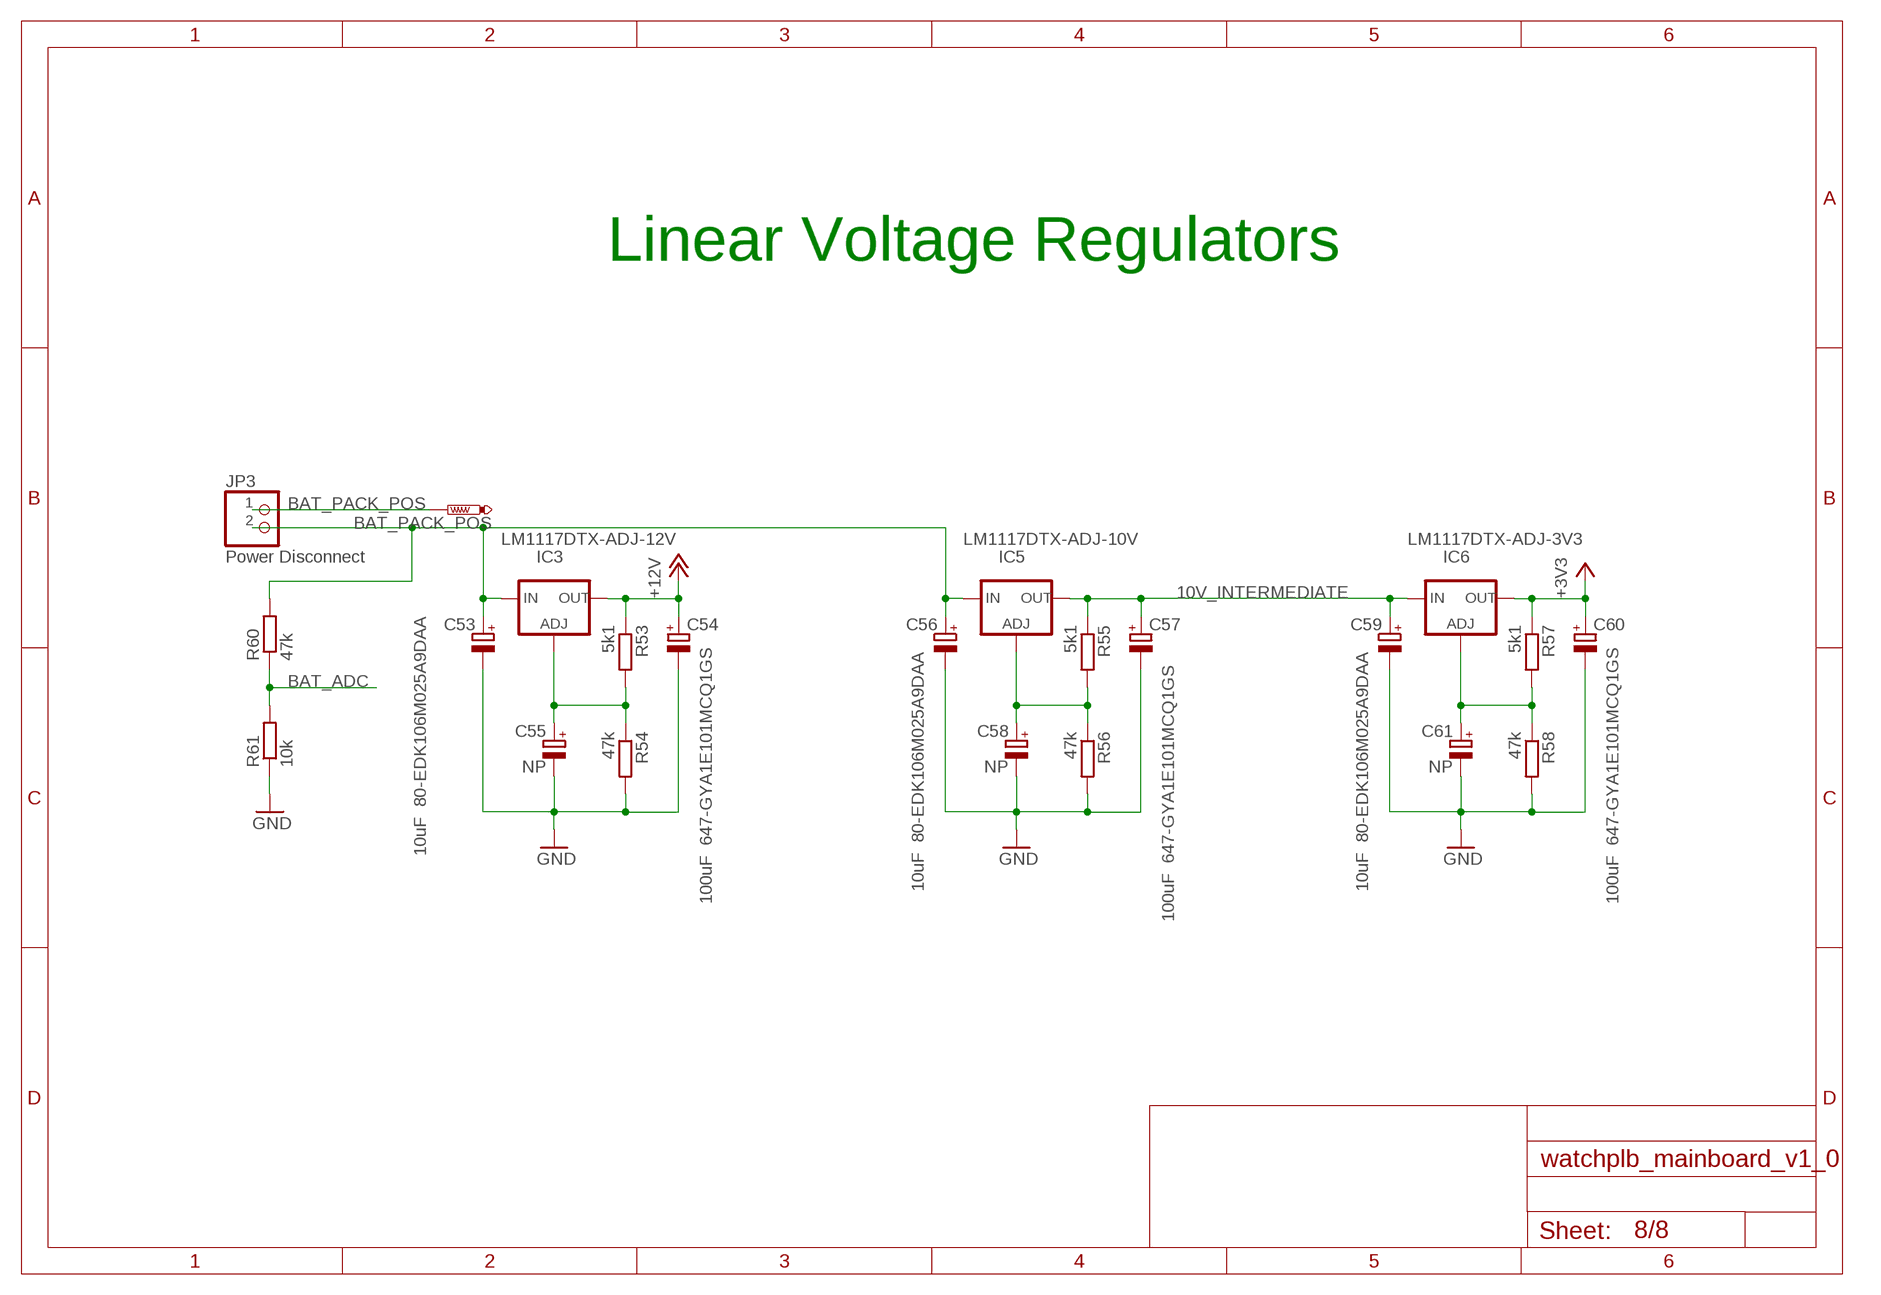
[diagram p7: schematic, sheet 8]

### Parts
BAT_PACK_POS  PTR1B1,27  [B1,27]
C53  10uF 80-EDK106M025A9DAA  CPOL-EUE  [PANASONIC_E]
C54  100uF 647-GYA1E101MCQ1GS  CPOL-EUE  [PANASONIC_E]
C55  NP  CPOL-EUE  [PANASONIC_E]
C56  10uF 80-EDK106M025A9DAA  CPOL-EUE  [PANASONIC_E]
C57  100uF 647-GYA1E101MCQ1GS  CPOL-EUE  [PANASONIC_E]
C58  NP  CPOL-EUE  [PANASONIC_E]
C59  10uF 80-EDK106M025A9DAA  CPOL-EUE  [PANASONIC_E]
C60  100uF 647-GYA1E101MCQ1GS  CPOL-EUE  [PANASONIC_E]
C61  NP  CPOL-EUE  [PANASONIC_E]
IC3  LM1117DTX-ADJ-12V  LM1117DTX-ADJ  [TO252]
IC5  LM1117DTX-ADJ-10V  LM1117DTX-ADJ  [TO252]
IC6  LM1117DTX-ADJ-3V3  LM1117DTX-ADJ  [TO252]
JP3  Power Disconnect  PINHD-1X2  [1X02]
R53  5k1  R-EU_M0805  [M0805]
R54  47k  R-EU_M0805  [M0805]
R55  5k1  R-EU_M0805  [M0805]
R56  47k  R-EU_M0805  [M0805]
R57  5k1  R-EU_M0805  [M0805]
R58  47k  R-EU_M0805  [M0805]
R60  47k  R-EU_M0805  [M0805]
R61  10k  R-EU_M0805  [M0805]

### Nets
10V_INTERMEDIATE: C57.+ C59.+ IC5.TAB(OUT) IC6.2(IN) R55.1
+3V3: C60.+ IC6.TAB(OUT) R57.1 ; also sheet 1,2,3,4,5,6
+12V: C54.+ IC3.TAB(OUT) R53.1 ; also sheet 2
BAT_ADC: R60.1 R61.2 ; also sheet 1
BAT_PACK_POS: BAT_PACK_POS.TP JP3.1 ; also sheet 5,7
GND: C53.- C54.- C55.- C56.- C57.- C58.- C59.- C60.- C61.- R54.2 R56.2 R58.2 R61.1 ; also sheet 1,2,3,4,5,6,7
N$84: C53.+ C56.+ IC3.2(IN) IC5.2(IN) JP3.2 R60.2
N$85: C55.+ IC3.1(ADJ) R53.2 R54.1
N$89: C58.+ IC5.1(ADJ) R55.2 R56.1
N$92: C61.+ IC6.1(ADJ) R57.2 R58.1

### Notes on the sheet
- Linear Voltage Regulators

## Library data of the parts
3V3 BAT_ADC BAT_PACK_POS BT_RX BT_TX BTN_1-BTN_4 BTN_NRST NRST_MCU RF_SIGNAL RF_SYSCLK SPI2_CLK SPI2_IRQ SPI2_MISO SPI2_MOSI SPI2_SEL_RFTX SWD_RXD SWD_TXD USB_DN USB_DP USB_ID = testpad:PTR1: TEST PIN
B1 B3-B7 = PCB4_Demoboard:B-EU_: EMI Filter
BAT CONFIG_INTERFACE_TEST_POINT PR0> = pinhead:PINHD-1X5: PIN HEADER
C4-C18 C20-C47 C49 = resistor:C-EU: CAPACITOR, European symbol
C19 = 12mhz osc:CSTCE8M00G52-R0; MANUFACTURER_PART_NUMBER: CSTCE8M00G52R0; VENDOR: Murata
C48 C51-C61 C63 = rcl:CPOL-EU: POLARIZED CAPACITOR, European symbol
D1 = diode:DIODE-: DIODE
D2-D5 D8 D9 = adafruit:DIODE: Diode
D6 D7 = diode-1:DIODE-: DIODE
D10 = diode:MBRS3*0T3: SCHOTTKY BARRIER RECTIFIER 3.0 AMPERES 20, 30, 40 VOLT
FB1 FB3 FB4 = SparkFun-Coils:FERRITE_BEAD: Ferrite Bead (blocks, cores, rings, chokes, etc.); PROD_ID: NDUC-13805; VALUE: 30O/1.8A
GPS> = pinhead:PINHD-1X8: PIN HEADER
IC1 = Hick:LT1513: Battery Charger Buck/Boost
IC2 = BM70BLES1FC2-0B03AA:BM70BLES1FC2-0B03AA: Bluetooth / 802.15.1 Modules Source: Datasheet; DESCRIPTION: Bluetooth / 802.15.1 Modules; HEIGHT: mm; MANUFACTURER_NAME: Microchip; MANUFACTURER_PART_NUMBER: BM70BLES1FC2-0B03AA
IC3 IC5 IC6 = lm1117:LM1117DTX-ADJ
IC4 = Hick:AX5031: AX5031 RF Transmitter 400-470MHz 800-940MHz
J1 J2 J4 = SparkFun-Connectors:USB_MICRO-B: USB Type Micro-B Connector Male/female and PTH/SMT variants SparkFun Products: SparkFun microB USB Breakout SparkFun USB microB Plug Breakout SparkFun ESP8266 Thing; PROD_ID: CONN-11752
J3 = SparkFun-Connectors:BNC: BNC Right Angle Connector; PROD_ID: LPA-12729; SF_ID: PRT-10550
JP2 JP3 = pinhead:PINHD-1X2: PIN HEADER
L1-L7 = SparkFun-Coils:INDUCTOR: Inductors; PROD_ID: NDUC-13076; VALUE: 3.3µH/±20%/450mA
L8 = CTX10-4A-R:CTX10-4A-R: POWER INDUCTOR; AVAILABILITY: Good; DESCRIPTION: Inductor Power Wirewound 10.53uH/42.11uH 25% 100KHz Amorphous Metal 4.67A/2.33A 20mOhm/81mOhm DCR T/R; MF: Eaton; MP: CTX10-4A-R; PACKAGE: Nonstandard Eaton; PRICE: 3.21 USD
LED1-LED12 = adafruit:LED: LED
Q1 = crystal:CRYSTAL: CRYSTAL; OC_FARNELL: unknown; OC_NEWARK: unknown
Q2 = transistor-npn:BC817*: NPN Transistor
Q3 Q7 = transistor-small-signal:BSS123: N-CHANNEL MOS FET
Q4 = adafruit:CRYSTAL: CRYSTAL; OC_FARNELL: unknown; OC_NEWARK: unknown
Q5 Q6 = CSD18534Q5A:CSD18534Q5A: 60V N-Channel NexFET Power? MOSFET 8-VSON-FET -55 to 150; AVAILABILITY: Good; DESCRIPTION: 60V N-Channel NexFET Power? MOSFET 8-VSON-FET -55 to 150; MF: Texas Instruments; MP: CSD18534Q5A; PACKAGE: VSON-8 Texas Instruments; PRICE: 0.61 USD
R3-R62 = resistor:R-EU_: RESISTOR, European symbol
S1-S5 = Hick:TL3305: OMRON SWITCH; MOUSER-NR: 612-TL3305AF260QG; MPN: TL3305
U1 = MCP111-XXXTO:MCP111-XXXXX/TO; MANUFACTURER_PART_NUMBER: MCP111XXXXXTO; VENDOR: Microchip
U2 = stm32l073rz_hoffentlich:STM32L0X3RL; MANUFACTURER_PART_NUMBER: stm32l0x3rl; VENDOR: STMicroelectronics
U3 = MCP2200-iSS:MCP2200-I/SS; MANUFACTURER_PART_NUMBER: mcp2200iss; VENDOR: Microchip
U4 = Texas Instruments_By_element14_Batch_1:TPD3E001DRLR: LOW-CAPACITANCE 3-CHANNEL ±15-kV ESD-PROTECTION ARRAY FOR HIGH-SPEED DATA INTERFACES; MPN: TPD3E001DRLR; OC_FARNELL: 1603422; OC_NEWARK: 41M5842; PACKAGE: SOT-5; SUPPLIER: Texas Instruments
U5 = chips:BQ77904: A battery protection chip with OV/UV/OT/UT; DIGIKEY: 296-44599-5-ND
U$2 = Hick:RA07H4047M

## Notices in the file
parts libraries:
SparkFun-Connectors: Licensing: Creative Commons ShareAlike 4.0 International - https://creativecommons.org/licenses/by-sa/4.0
